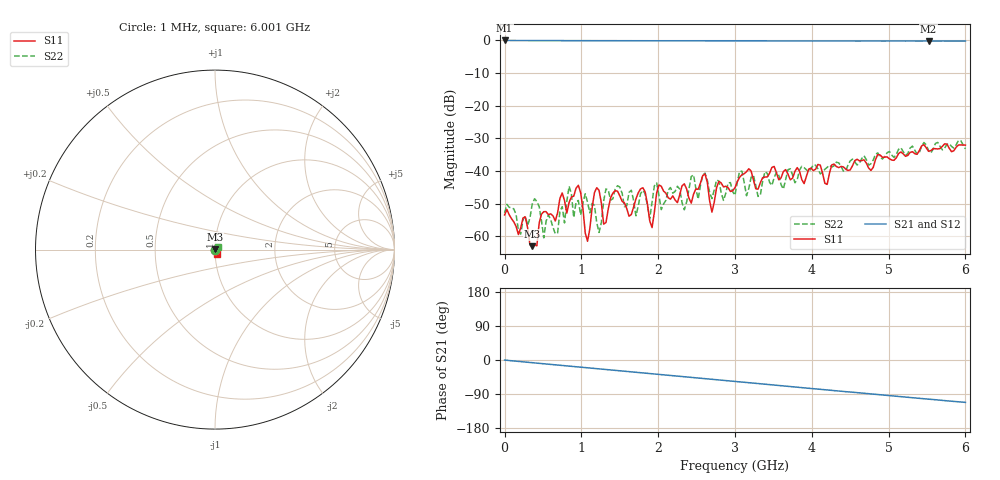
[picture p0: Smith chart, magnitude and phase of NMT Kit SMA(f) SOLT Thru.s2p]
! NMT Kit SMA(f) typ SOLT V1 - Thru s2p data
! Ref Plane 0 mm
#  MHz  S  RI  R  50
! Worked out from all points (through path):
!   201 points, 1 MHz to 6.001 GHz, reference 50 ohm
!   highest |S21| = 0.00 dB at 1 MHz (marker M1); lowest = -0.2 dB at 5.521 GHz (marker M2)
!   group delay of S21, straight-line fit = 51.8 ps
!   lowest |S11| = -63.1 dB at 361 MHz (marker M3), VSWR 1.00, Z = 50 + j0.0591 ohm
!   |S11| at or under -10 dB: start of sweep to end of sweep
!   |S22| runs from -60.5 to -30.7 dB; largest |S21 - S12| = 0.033
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1  0.00212 0.000184  1 -0.00105  0.9995 0.00436  0.00227 0.000201
211  0.00128 -0.00042  0.9938 -0.0751  0.9949 -0.0443  0.00107 -0.000129
361  -0.000381 0.000591  0.9876 -0.1234  0.9911 -0.0937  0.00184 -0.0025
511  -0.00216 -0.000987  0.98 -0.1719  0.984 -0.1418  0.0009 -0.00028
781  -0.00185 -0.003  0.96 -0.2569  0.9662 -0.2282  -0.000289 0.00157
841  -0.00184 0.00274  0.9545 -0.2757  0.9615 -0.2472  -0.00495 0.0031
901  -0.00393 0.00119  0.9484 -0.2943  0.9563 -0.2663  -0.0013 0.00143
1021  -0.0026 0.000476  0.9355 -0.3311  0.9445 -0.3038  0.00168 -0.00274
1081  -0.000553 0.000627  0.9286 -0.3492  0.9381 -0.3221  0.00287 -0.00165
1201  0.00287 0.00473  0.9139 -0.3853  0.9241 -0.359  -0.00127 -0.00098
1291  0.00101 0.00115  0.9019 -0.412  0.9128 -0.3856  -0.00342 0.00062
1801  0.00466 0.00298  0.8193 -0.5551  0.8353 -0.5287  -0.00162 -0.00477
1921  -0.000921 0.000994  0.7966 -0.5863  0.8134 -0.5613  0.00324 -0.000834
2011  -0.00109 0.00601  0.7787 -0.6093  0.7966 -0.5854  0.00273 0.0032
2341  -0.00402 0.00491  0.7079 -0.6882  0.7285 -0.6674  -0.00249 -0.0005
2611  -0.00213 0.00872  0.6442 -0.7476  0.6666 -0.7287  0.00926 0.000518
2701  0.00228 0.000552  0.6228 -0.7655  0.6447 -0.7479  0.00158 0.00342
3001  0.00328 -0.00447  0.5439 -0.8224  0.5683 -0.8077  -0.00149 0.00397
4021  0.00531 -0.00865  0.2444 -0.9519  0.2692 -0.9464  0.0016 0.0123
5011  0.00961 -0.012  -0.0685 -0.9814  -0.0423 -0.9835  0.00495 0.0193
5521  0.00949 -0.0176  -0.2259 -0.9528  -0.2021 -0.9641  0.0112 0.0172
6001  0.00983 -0.0229  -0.3642 -0.9091  -0.3461 -0.9222  0.0171 0.0136
